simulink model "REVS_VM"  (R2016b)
settings: Solver=ode3  StartTime=REVS.sim_start_time_secs  StopTime=Inf  FixedStep=REVS.sim_step_time_secs  MaxStep=REVS.sim_step_time_secs  EnableMultiTasking=on
StopFcn:
  | postproc_datalog;
  | postproc_audit;
  | postproc_result;
model workspace (MATLAB code in the model file):
  other statements: REVS_setup_variants
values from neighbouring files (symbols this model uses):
  accessory = class_accessory_data    [class_test_data.m]
  battery = class_battery_data    [class_accessory_data.m]    (also in class_REVS_electric.m = class_REVS_battery)
  brake = struct(	'max_torque_Nm',[], 						'proportion_norm',1.0, 						'inertia_kgm2',0.0)    [class_REVS_drive_axle.m]
  engine = class_engine_data    [class_test_data.m]
  final_drive = struct(	'gear_ratio',[], 								'efficiency_norm',[], 								'inertia_kgm2',[] )    [class_REVS_drive_axle.m]
  gear = class_REVS_gearbox    [class_REVS_AT_transmission.m]
  tire = struct(	'radius_m',[], 						'rolling_resistance_coefficient',0, 						'vehicle_weight_norm',1.0,  						'wheel_slip_torque_Nm',[],  						'inertia_kgm2',0.0)    [class_REVS_drive_axle.m]
  torque_converter = class_REVS_torque_converter    [class_REVS_AT_transmission.m]
  transmission = class_transmission_data    [class_test_data.m]
  vehicle = class_vehicle_data    [class_test_data.m]
undefined symbols (not defined in the file or in its folder): alternator, ambient, controls, convert, DelayTimeSecs, drive_cycle, driver, electric, gear_strategy, InitialCondition, InitialValue, LoadSource, LookupStructure, MultiplyPosInputs, Normalize, NumPhases, REVS, SpeedSource, starter, tableshift, UpperSaturationLimit, Value, VerboseLevel, VerboseSignal
libraries: simulink x153
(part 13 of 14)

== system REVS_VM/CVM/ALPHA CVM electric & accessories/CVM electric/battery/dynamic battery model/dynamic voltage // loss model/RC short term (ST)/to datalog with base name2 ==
  Var : Inport
  Constant : Constant  Value=VerboseSignal
  Constant1 : Constant  Value=VerboseLevel
  Relational Operator : RelationalOperator  OutDataTypeStr=boolean  ZeroCross=off
  Subsystem : Subsystem
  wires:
  Constant1/1 -> Relational Operator/2
  Relational Operator/1 -> Subsystem/Enable
  Constant/1 -> Relational Operator/1
  Var/1 -> Subsystem/1(Var)

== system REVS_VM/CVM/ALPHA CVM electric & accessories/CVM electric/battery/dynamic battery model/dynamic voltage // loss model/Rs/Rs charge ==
  bus : Inport
  Bus Selector : BusSelector  OutputSignals=gb.gb_cmd_gear,gb_spd_in_radps,ctrl.gb_line_press_bar
  Lookup : Lookup_n-D  NumberOfTableDimensions=10  BreakpointsForDimension1=LookupStructure.axis_1.breakpoints  BreakpointsForDimension2=LookupStructure.axis_2.breakpoints  BreakpointsForDimension3=LookupStructure.axis_3.breakpoints  BreakpointsForDimension4=LookupStructure.axis_4.breakpoints  BreakpointsForDimension5=LookupStructure.axis_5.breakpoints  BreakpointsForDimension6=LookupStructure.axis_6.breakpoints  BreakpointsForDimension7=LookupStructure.axis_7.breakpoints  BreakpointsForDimension8=LookupStructure.axis_8.breakpoints  BreakpointsForDimension9=LookupStructure.axis_9.breakpoints  BreakpointsForDimension10=LookupStructure.axis_10.breakpoints  IndexSearchMethod=Linear search  BeginIndexSearchUsingPreviousIndexResult=on  Table=LookupStructure.table  InternalRulePriority=Speed  RndMeth=Simplest  SupportTunableTableSize=on  MaximumIndicesForEachDimension=LookupStructure.table_size
  out : Outport
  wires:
  bus/1 -> Bus Selector/1
  Lookup/1 -> out/1

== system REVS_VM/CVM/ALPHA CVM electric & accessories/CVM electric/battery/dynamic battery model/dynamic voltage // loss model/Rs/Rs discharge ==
  bus : Inport
  Bus Selector : BusSelector  OutputSignals=gb.gb_cmd_gear,gb_spd_in_radps,ctrl.gb_line_press_bar
  Lookup : Lookup_n-D  NumberOfTableDimensions=10  BreakpointsForDimension1=LookupStructure.axis_1.breakpoints  BreakpointsForDimension2=LookupStructure.axis_2.breakpoints  BreakpointsForDimension3=LookupStructure.axis_3.breakpoints  BreakpointsForDimension4=LookupStructure.axis_4.breakpoints  BreakpointsForDimension5=LookupStructure.axis_5.breakpoints  BreakpointsForDimension6=LookupStructure.axis_6.breakpoints  BreakpointsForDimension7=LookupStructure.axis_7.breakpoints  BreakpointsForDimension8=LookupStructure.axis_8.breakpoints  BreakpointsForDimension9=LookupStructure.axis_9.breakpoints  BreakpointsForDimension10=LookupStructure.axis_10.breakpoints  IndexSearchMethod=Linear search  BeginIndexSearchUsingPreviousIndexResult=on  Table=LookupStructure.table  InternalRulePriority=Speed  RndMeth=Simplest  SupportTunableTableSize=on  MaximumIndicesForEachDimension=LookupStructure.table_size
  out : Outport
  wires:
  bus/1 -> Bus Selector/1
  Lookup/1 -> out/1

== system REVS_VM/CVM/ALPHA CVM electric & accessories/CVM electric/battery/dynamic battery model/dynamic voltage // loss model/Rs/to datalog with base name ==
  Var : Inport
  Constant : Constant  Value=VerboseSignal
  Constant1 : Constant  Value=VerboseLevel
  Relational Operator : RelationalOperator  OutDataTypeStr=boolean  ZeroCross=off
  Subsystem : Subsystem
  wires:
  Constant1/1 -> Relational Operator/2
  Relational Operator/1 -> Subsystem/Enable
  Constant/1 -> Relational Operator/1
  Var/1 -> Subsystem/1(Var)

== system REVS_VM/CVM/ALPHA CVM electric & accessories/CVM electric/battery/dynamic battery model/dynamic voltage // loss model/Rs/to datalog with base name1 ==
  Var : Inport
  Constant : Constant  Value=VerboseSignal
  Constant1 : Constant  Value=VerboseLevel
  Relational Operator : RelationalOperator  OutDataTypeStr=boolean  ZeroCross=off
  Subsystem : Subsystem
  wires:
  Constant1/1 -> Relational Operator/2
  Relational Operator/1 -> Subsystem/Enable
  Constant/1 -> Relational Operator/1
  Var/1 -> Subsystem/1(Var)

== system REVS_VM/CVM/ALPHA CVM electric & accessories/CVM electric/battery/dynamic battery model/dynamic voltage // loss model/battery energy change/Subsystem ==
  In1 : Inport
  Enable : EnablePort
  To Workspace : ToWorkspace  VariableName=audit__elec__battery__energy_delta_kJ  SampleTime=-1
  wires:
  In1/1 -> To Workspace/1

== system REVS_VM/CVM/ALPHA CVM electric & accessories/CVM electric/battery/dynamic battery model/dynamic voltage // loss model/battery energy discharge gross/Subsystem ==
  In1 : Inport
  Enable : EnablePort
  To Workspace : ToWorkspace  VariableName=audit__elec__battery__discharge_gross_kJ  SampleTime=-1
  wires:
  In1/1 -> To Workspace/1

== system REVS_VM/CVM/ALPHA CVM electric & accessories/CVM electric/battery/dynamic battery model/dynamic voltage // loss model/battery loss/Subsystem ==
  In1 : Inport
  Enable : EnablePort
  To Workspace : ToWorkspace  VariableName=audit__elec__battery__loss_kJ  SampleTime=-1
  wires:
  In1/1 -> To Workspace/1

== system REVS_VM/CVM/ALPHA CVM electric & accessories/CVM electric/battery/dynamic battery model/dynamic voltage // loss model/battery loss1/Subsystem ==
  In1 : Inport
  Enable : EnablePort
  To Workspace : ToWorkspace  VariableName=audit__elec__battery__OCV  SampleTime=-1
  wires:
  In1/1 -> To Workspace/1

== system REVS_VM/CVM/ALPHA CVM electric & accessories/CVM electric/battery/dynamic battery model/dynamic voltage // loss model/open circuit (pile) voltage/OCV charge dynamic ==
  bus : Inport
  Bus Selector : BusSelector  OutputSignals=gb.gb_cmd_gear,gb_spd_in_radps,ctrl.gb_line_press_bar
  Lookup : Lookup_n-D  NumberOfTableDimensions=10  BreakpointsForDimension1=LookupStructure.axis_1.breakpoints  BreakpointsForDimension2=LookupStructure.axis_2.breakpoints  BreakpointsForDimension3=LookupStructure.axis_3.breakpoints  BreakpointsForDimension4=LookupStructure.axis_4.breakpoints  BreakpointsForDimension5=LookupStructure.axis_5.breakpoints  BreakpointsForDimension6=LookupStructure.axis_6.breakpoints  BreakpointsForDimension7=LookupStructure.axis_7.breakpoints  BreakpointsForDimension8=LookupStructure.axis_8.breakpoints  BreakpointsForDimension9=LookupStructure.axis_9.breakpoints  BreakpointsForDimension10=LookupStructure.axis_10.breakpoints  IndexSearchMethod=Linear search  BeginIndexSearchUsingPreviousIndexResult=on  Table=LookupStructure.table  InternalRulePriority=Speed  RndMeth=Simplest  SupportTunableTableSize=on  MaximumIndicesForEachDimension=LookupStructure.table_size
  out : Outport
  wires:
  bus/1 -> Bus Selector/1
  Lookup/1 -> out/1

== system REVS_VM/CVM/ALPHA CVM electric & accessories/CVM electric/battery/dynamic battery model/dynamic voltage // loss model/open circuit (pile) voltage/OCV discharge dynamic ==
  bus : Inport
  Bus Selector : BusSelector  OutputSignals=gb.gb_cmd_gear,gb_spd_in_radps,ctrl.gb_line_press_bar
  Lookup : Lookup_n-D  NumberOfTableDimensions=10  BreakpointsForDimension1=LookupStructure.axis_1.breakpoints  BreakpointsForDimension2=LookupStructure.axis_2.breakpoints  BreakpointsForDimension3=LookupStructure.axis_3.breakpoints  BreakpointsForDimension4=LookupStructure.axis_4.breakpoints  BreakpointsForDimension5=LookupStructure.axis_5.breakpoints  BreakpointsForDimension6=LookupStructure.axis_6.breakpoints  BreakpointsForDimension7=LookupStructure.axis_7.breakpoints  BreakpointsForDimension8=LookupStructure.axis_8.breakpoints  BreakpointsForDimension9=LookupStructure.axis_9.breakpoints  BreakpointsForDimension10=LookupStructure.axis_10.breakpoints  IndexSearchMethod=Linear search  BeginIndexSearchUsingPreviousIndexResult=on  Table=LookupStructure.table  InternalRulePriority=Speed  RndMeth=Simplest  SupportTunableTableSize=on  MaximumIndicesForEachDimension=LookupStructure.table_size
  out : Outport
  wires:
  bus/1 -> Bus Selector/1
  Lookup/1 -> out/1

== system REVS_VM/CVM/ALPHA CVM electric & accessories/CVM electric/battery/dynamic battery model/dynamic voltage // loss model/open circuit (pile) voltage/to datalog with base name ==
  Var : Inport
  Constant : Constant  Value=VerboseSignal
  Constant1 : Constant  Value=VerboseLevel
  Relational Operator : RelationalOperator  OutDataTypeStr=boolean  ZeroCross=off
  Subsystem : Subsystem
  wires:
  Constant1/1 -> Relational Operator/2
  Relational Operator/1 -> Subsystem/Enable
  Constant/1 -> Relational Operator/1
  Var/1 -> Subsystem/1(Var)

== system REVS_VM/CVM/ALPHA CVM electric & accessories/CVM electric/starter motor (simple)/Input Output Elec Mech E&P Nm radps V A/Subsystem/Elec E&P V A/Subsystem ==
  volts_V : Inport
  curr_A : Inport  Port=2
  Enable : EnablePort  ZeroCross=off
  Elec Energy V A : Subsystem  TreatAsAtomicUnit=on
  amps_to_workspace : ToWorkspace  VariableName=audit__elec__starter__input_Amps  SampleTime=-1
  energy_to_workspace : ToWorkspace  VariableName=audit__elec__starter__input_kJ  SampleTime=-1
  neg_energy_to_workspace : ToWorkspace  VariableName=audit__elec__starter__input_neg_kJ  SampleTime=-1
  pos_energy_to_workspace : ToWorkspace  VariableName=audit__elec__starter__input_pos_kJ  SampleTime=-1
  power_to_workspace : ToWorkspace  VariableName=audit__elec__starter__input_kW  SampleTime=-1
  volts_to_workspace : ToWorkspace  VariableName=audit__elec__starter__input_Volts  SampleTime=-1
  pos_kJ : Outport  InitialOutput=0
  neg_kJ : Outport  Port=2  InitialOutput=0
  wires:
  Elec Energy V A/3(neg_kJ) -> neg_kJ/1, neg_energy_to_workspace/1
  Elec Energy V A/4(pwr_kW) -> power_to_workspace/1
  Elec Energy V A/2("pos_kJ ") -> pos_kJ/1, pos_energy_to_workspace/1
  Elec Energy V A/1("total_kJ ") -> energy_to_workspace/1
  volts_V/1 -> volts_to_workspace/1, Elec Energy V A/1(volts_V)
  curr_A/1 -> amps_to_workspace/1, Elec Energy V A/2(curr_A)

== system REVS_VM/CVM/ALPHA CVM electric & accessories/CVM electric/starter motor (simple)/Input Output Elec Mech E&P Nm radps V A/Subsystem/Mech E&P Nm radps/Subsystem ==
  " trq_Nm" : Inport
  spd_radps : Inport  Port=2
  iner_kgm2 : Inport  Port=3
  Enable : EnablePort  ZeroCross=off
  KE_to_workspace : ToWorkspace  VariableName=audit__mech__starter__output_KE_kJ  SampleTime=-1
  Mech Energy Nm radps : Subsystem  TreatAsAtomicUnit=on
  Mult : Product  Inputs=**
  Square : Math  Operator=square
  energy_to_workspace : ToWorkspace  VariableName=audit__mech__starter__output_kJ  SampleTime=-1
  inertia_to_workspace : ToWorkspace  VariableName=audit__mech__starter__output_kgm2  SampleTime=-1
  neg_energy_to_workspace : ToWorkspace  VariableName=audit__mech__starter__output_neg_kJ  SampleTime=-1
  one half : Gain  Gain=0.5/1000
  pos_energy_to_workspace : ToWorkspace  VariableName=audit__mech__starter__output_pos_kJ  SampleTime=-1
  power_to_workspace : ToWorkspace  VariableName=audit__mech__starter__output_kW  SampleTime=-1
  speed_to_workspace : ToWorkspace  VariableName=audit__mech__starter__output_radps  SampleTime=-1
  torque_to_workspace : ToWorkspace  VariableName=audit__mech__starter__output_Nm  SampleTime=-1
  pos_kJ : Outport  InitialOutput=0
  neg_kJ : Outport  Port=2  InitialOutput=0
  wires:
  Mult/1 -> one half/1
  Square/1 -> Mult/1
  one half/1 -> KE_to_workspace/1
  Mech Energy Nm radps/4(pwr_kW) -> power_to_workspace/1
  Mech Energy Nm radps/1("total_kJ ") -> energy_to_workspace/1
  iner_kgm2/1 -> inertia_to_workspace/1, Mult/2
  spd_radps/1 -> Mech Energy Nm radps/2(spd_radps), speed_to_workspace/1, Square/1
  " trq_Nm"/1 -> Mech Energy Nm radps/1(trq_Nm), torque_to_workspace/1
  Mech Energy Nm radps/2("pos_kJ ") -> pos_kJ/1, pos_energy_to_workspace/1
  Mech Energy Nm radps/3(neg_kJ) -> neg_energy_to_workspace/1, neg_kJ/1

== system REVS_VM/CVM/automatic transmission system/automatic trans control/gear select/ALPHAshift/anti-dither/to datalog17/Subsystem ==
  In1 : Inport
  Enable : EnablePort
  To Workspace : ToWorkspace  VariableName=datalog__ALPHAshift__filtered_desired_gear_num  SampleTime=-1
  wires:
  In1/1 -> To Workspace/1

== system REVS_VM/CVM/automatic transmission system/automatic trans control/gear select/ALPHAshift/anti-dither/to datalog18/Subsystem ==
  In1 : Inport
  Enable : EnablePort
  To Workspace : ToWorkspace  VariableName=datalog__ALPHAshift__raw_desired_gear_num  SampleTime=-1
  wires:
  In1/1 -> To Workspace/1

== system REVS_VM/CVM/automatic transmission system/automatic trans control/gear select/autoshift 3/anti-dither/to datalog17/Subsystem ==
  In1 : Inport
  Enable : EnablePort
  To Workspace : ToWorkspace  VariableName=datalog__autoshift3__filtered_desired_gear_num  SampleTime=-1
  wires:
  In1/1 -> To Workspace/1

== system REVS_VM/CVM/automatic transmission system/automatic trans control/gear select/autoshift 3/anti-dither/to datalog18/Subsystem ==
  In1 : Inport
  Enable : EnablePort
  To Workspace : ToWorkspace  VariableName=datalog__autoshift3__raw_desired_gear_num  SampleTime=-1
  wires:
  In1/1 -> To Workspace/1

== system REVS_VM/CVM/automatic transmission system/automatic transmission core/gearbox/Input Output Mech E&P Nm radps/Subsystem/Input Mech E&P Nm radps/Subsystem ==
  " trq_Nm" : Inport
  spd_radps : Inport  Port=2
  iner_kgm2 : Inport  Port=3
  Enable : EnablePort  ZeroCross=off
  KE_to_workspace : ToWorkspace  VariableName=audit__mech__gearbox__input_KE_kJ  SampleTime=-1
  Mech Energy Nm radps : Subsystem  TreatAsAtomicUnit=on
  Mult : Product  Inputs=**
  Square : Math  Operator=square
  energy_to_workspace : ToWorkspace  VariableName=audit__mech__gearbox__input_kJ  SampleTime=-1
  inertia_to_workspace : ToWorkspace  VariableName=audit__mech__gearbox__input_kgm2  SampleTime=-1
  neg_energy_to_workspace : ToWorkspace  VariableName=audit__mech__gearbox__input_neg_kJ  SampleTime=-1
  one half : Gain  Gain=0.5/1000
  pos_energy_to_workspace : ToWorkspace  VariableName=audit__mech__gearbox__input_pos_kJ  SampleTime=-1
  power_to_workspace : ToWorkspace  VariableName=audit__mech__gearbox__input_kW  SampleTime=-1
  speed_to_workspace : ToWorkspace  VariableName=audit__mech__gearbox__input_radps  SampleTime=-1
  torque_to_workspace : ToWorkspace  VariableName=audit__mech__gearbox__input_Nm  SampleTime=-1
  pos_kJ : Outport  InitialOutput=0
  neg_kJ : Outport  Port=2  InitialOutput=0
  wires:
  Mult/1 -> one half/1
  Square/1 -> Mult/1
  one half/1 -> KE_to_workspace/1
  Mech Energy Nm radps/4(pwr_kW) -> power_to_workspace/1
  Mech Energy Nm radps/1("total_kJ ") -> energy_to_workspace/1
  iner_kgm2/1 -> inertia_to_workspace/1, Mult/2
  spd_radps/1 -> Mech Energy Nm radps/2(spd_radps), speed_to_workspace/1, Square/1
  " trq_Nm"/1 -> Mech Energy Nm radps/1(trq_Nm), torque_to_workspace/1
  Mech Energy Nm radps/2("pos_kJ ") -> pos_kJ/1, pos_energy_to_workspace/1
  Mech Energy Nm radps/3(neg_kJ) -> neg_energy_to_workspace/1, neg_kJ/1

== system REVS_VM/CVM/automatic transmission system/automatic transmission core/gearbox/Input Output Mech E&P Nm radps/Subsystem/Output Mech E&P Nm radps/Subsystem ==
  " trq_Nm" : Inport
  spd_radps : Inport  Port=2
  iner_kgm2 : Inport  Port=3
  Enable : EnablePort  ZeroCross=off
  KE_to_workspace : ToWorkspace  VariableName=audit__mech__gearbox__output_KE_kJ  SampleTime=-1
  Mech Energy Nm radps : Subsystem  TreatAsAtomicUnit=on
  Mult : Product  Inputs=**
  Square : Math  Operator=square
  energy_to_workspace : ToWorkspace  VariableName=audit__mech__gearbox__output_kJ  SampleTime=-1
  inertia_to_workspace : ToWorkspace  VariableName=audit__mech__gearbox__output_kgm2  SampleTime=-1
  neg_energy_to_workspace : ToWorkspace  VariableName=audit__mech__gearbox__output_neg_kJ  SampleTime=-1
  one half : Gain  Gain=0.5/1000
  pos_energy_to_workspace : ToWorkspace  VariableName=audit__mech__gearbox__output_pos_kJ  SampleTime=-1
  power_to_workspace : ToWorkspace  VariableName=audit__mech__gearbox__output_kW  SampleTime=-1
  speed_to_workspace : ToWorkspace  VariableName=audit__mech__gearbox__output_radps  SampleTime=-1
  torque_to_workspace : ToWorkspace  VariableName=audit__mech__gearbox__output_Nm  SampleTime=-1
  pos_kJ : Outport  InitialOutput=0
  neg_kJ : Outport  Port=2  InitialOutput=0
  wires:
  Mult/1 -> one half/1
  Square/1 -> Mult/1
  one half/1 -> KE_to_workspace/1
  Mech Energy Nm radps/4(pwr_kW) -> power_to_workspace/1
  Mech Energy Nm radps/1("total_kJ ") -> energy_to_workspace/1
  iner_kgm2/1 -> inertia_to_workspace/1, Mult/2
  spd_radps/1 -> Mech Energy Nm radps/2(spd_radps), speed_to_workspace/1, Square/1
  " trq_Nm"/1 -> Mech Energy Nm radps/1(trq_Nm), torque_to_workspace/1
  Mech Energy Nm radps/2("pos_kJ ") -> pos_kJ/1, pos_energy_to_workspace/1
  Mech Energy Nm radps/3(neg_kJ) -> neg_energy_to_workspace/1, neg_kJ/1

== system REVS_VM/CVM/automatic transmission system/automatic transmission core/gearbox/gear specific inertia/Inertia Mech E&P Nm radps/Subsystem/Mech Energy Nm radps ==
  trq_Nm : Inport
  spd_radps : Inport  Port=2
  Gain : Gain  Gain=-1
  Integrator : Integrator  ZeroCross=off
  Integrator1 : Integrator  ZeroCross=off
  Integrator2 : Integrator  ZeroCross=off
  Mux : Mux  Inputs=2
  Neg : Fcn  Expr=u(1)*(u(1) <= 0)
  Pos : Fcn  Expr=u(1)*(u(1) >= 0)
  calc_Power_kW : Fcn  Expr=u(1)*u(2)/1000
  "total_kJ " : Outport
  "pos_kJ " : Outport  Port=2
  neg_kJ : Outport  Port=3
  pwr_kW : Outport  Port=4
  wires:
  calc_Power_kW/1 -> Pos/1, Neg/1, pwr_kW/1, Integrator/1
  Gain/1 -> neg_kJ/1
  Integrator1/1 -> "pos_kJ "/1
  Integrator2/1 -> Gain/1
  Neg/1 -> Integrator2/1
  Pos/1 -> Integrator1/1
  spd_radps/1 -> Mux/2
  trq_Nm/1 -> Mux/1
  Mux/1 -> calc_Power_kW/1
  Integrator/1 -> "total_kJ "/1

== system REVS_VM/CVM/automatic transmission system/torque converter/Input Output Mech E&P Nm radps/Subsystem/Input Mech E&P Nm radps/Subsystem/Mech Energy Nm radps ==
  trq_Nm : Inport
  spd_radps : Inport  Port=2
  Gain : Gain  Gain=-1
  Integrator : Integrator  ZeroCross=off
  Integrator1 : Integrator  ZeroCross=off
  Integrator2 : Integrator  ZeroCross=off
  Mux : Mux  Inputs=2
  Neg : Fcn  Expr=u(1)*(u(1) <= 0)
  Pos : Fcn  Expr=u(1)*(u(1) >= 0)
  calc_Power_kW : Fcn  Expr=u(1)*u(2)/1000
  "total_kJ " : Outport
  "pos_kJ " : Outport  Port=2
  neg_kJ : Outport  Port=3
  pwr_kW : Outport  Port=4
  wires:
  calc_Power_kW/1 -> Pos/1, Neg/1, pwr_kW/1, Integrator/1
  Gain/1 -> neg_kJ/1
  Integrator1/1 -> "pos_kJ "/1
  Integrator2/1 -> Gain/1
  Neg/1 -> Integrator2/1
  Pos/1 -> Integrator1/1
  spd_radps/1 -> Mux/2
  trq_Nm/1 -> Mux/1
  Mux/1 -> calc_Power_kW/1
  Integrator/1 -> "total_kJ "/1

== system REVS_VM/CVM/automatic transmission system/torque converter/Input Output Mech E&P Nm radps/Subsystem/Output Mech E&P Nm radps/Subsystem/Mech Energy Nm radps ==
  trq_Nm : Inport
  spd_radps : Inport  Port=2
  Gain : Gain  Gain=-1
  Integrator : Integrator  ZeroCross=off
  Integrator1 : Integrator  ZeroCross=off
  Integrator2 : Integrator  ZeroCross=off
  Mux : Mux  Inputs=2
  Neg : Fcn  Expr=u(1)*(u(1) <= 0)
  Pos : Fcn  Expr=u(1)*(u(1) >= 0)
  calc_Power_kW : Fcn  Expr=u(1)*u(2)/1000
  "total_kJ " : Outport
  "pos_kJ " : Outport  Port=2
  neg_kJ : Outport  Port=3
  pwr_kW : Outport  Port=4
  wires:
  calc_Power_kW/1 -> Pos/1, Neg/1, pwr_kW/1, Integrator/1
  Gain/1 -> neg_kJ/1
  Integrator1/1 -> "pos_kJ "/1
  Integrator2/1 -> Gain/1
  Neg/1 -> Integrator2/1
  Pos/1 -> Integrator1/1
  spd_radps/1 -> Mux/2
  trq_Nm/1 -> Mux/1
  Mux/1 -> calc_Power_kW/1
  Integrator/1 -> "total_kJ "/1

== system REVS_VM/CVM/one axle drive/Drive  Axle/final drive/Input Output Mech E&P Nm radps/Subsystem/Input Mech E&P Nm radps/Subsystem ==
  " trq_Nm" : Inport
  spd_radps : Inport  Port=2
  iner_kgm2 : Inport  Port=3
  Enable : EnablePort  ZeroCross=off
  KE_to_workspace : ToWorkspace  VariableName=audit__mech__drive_axle1__final_drive__input_KE_kJ  SampleTime=-1
  Mech Energy Nm radps : Subsystem  TreatAsAtomicUnit=on
  Mult : Product  Inputs=**
  Square : Math  Operator=square
  energy_to_workspace : ToWorkspace  VariableName=audit__mech__drive_axle1__final_drive__input_kJ  SampleTime=-1
  inertia_to_workspace : ToWorkspace  VariableName=audit__mech__drive_axle1__final_drive__input_kgm2  SampleTime=-1
  neg_energy_to_workspace : ToWorkspace  VariableName=audit__mech__drive_axle1__final_drive__input_neg_kJ  SampleTime=-1
  one half : Gain  Gain=0.5/1000
  pos_energy_to_workspace : ToWorkspace  VariableName=audit__mech__drive_axle1__final_drive__input_pos_kJ  SampleTime=-1
  power_to_workspace : ToWorkspace  VariableName=audit__mech__drive_axle1__final_drive__input_kW  SampleTime=-1
  speed_to_workspace : ToWorkspace  VariableName=audit__mech__drive_axle1__final_drive__input_radps  SampleTime=-1
  torque_to_workspace : ToWorkspace  VariableName=audit__mech__drive_axle1__final_drive__input_Nm  SampleTime=-1
  pos_kJ : Outport  InitialOutput=0
  neg_kJ : Outport  Port=2  InitialOutput=0
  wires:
  Mult/1 -> one half/1
  Square/1 -> Mult/1
  one half/1 -> KE_to_workspace/1
  Mech Energy Nm radps/4(pwr_kW) -> power_to_workspace/1
  Mech Energy Nm radps/1("total_kJ ") -> energy_to_workspace/1
  iner_kgm2/1 -> inertia_to_workspace/1, Mult/2
  spd_radps/1 -> Mech Energy Nm radps/2(spd_radps), speed_to_workspace/1, Square/1
  " trq_Nm"/1 -> Mech Energy Nm radps/1(trq_Nm), torque_to_workspace/1
  Mech Energy Nm radps/2("pos_kJ ") -> pos_kJ/1, pos_energy_to_workspace/1
  Mech Energy Nm radps/3(neg_kJ) -> neg_energy_to_workspace/1, neg_kJ/1

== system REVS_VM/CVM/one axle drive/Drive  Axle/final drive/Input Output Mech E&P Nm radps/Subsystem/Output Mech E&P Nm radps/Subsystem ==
  " trq_Nm" : Inport
  spd_radps : Inport  Port=2
  iner_kgm2 : Inport  Port=3
  Enable : EnablePort  ZeroCross=off
  KE_to_workspace : ToWorkspace  VariableName=audit__mech__drive_axle1__final_drive__output_KE_kJ  SampleTime=-1
  Mech Energy Nm radps : Subsystem  TreatAsAtomicUnit=on
  Mult : Product  Inputs=**
  Square : Math  Operator=square
  energy_to_workspace : ToWorkspace  VariableName=audit__mech__drive_axle1__final_drive__output_kJ  SampleTime=-1
  inertia_to_workspace : ToWorkspace  VariableName=audit__mech__drive_axle1__final_drive__output_kgm2  SampleTime=-1
  neg_energy_to_workspace : ToWorkspace  VariableName=audit__mech__drive_axle1__final_drive__output_neg_kJ  SampleTime=-1
  one half : Gain  Gain=0.5/1000
  pos_energy_to_workspace : ToWorkspace  VariableName=audit__mech__drive_axle1__final_drive__output_pos_kJ  SampleTime=-1
  power_to_workspace : ToWorkspace  VariableName=audit__mech__drive_axle1__final_drive__output_kW  SampleTime=-1
  speed_to_workspace : ToWorkspace  VariableName=audit__mech__drive_axle1__final_drive__output_radps  SampleTime=-1
  torque_to_workspace : ToWorkspace  VariableName=audit__mech__drive_axle1__final_drive__output_Nm  SampleTime=-1
  pos_kJ : Outport  InitialOutput=0
  neg_kJ : Outport  Port=2  InitialOutput=0
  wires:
  Mult/1 -> one half/1
  Square/1 -> Mult/1
  one half/1 -> KE_to_workspace/1
  Mech Energy Nm radps/4(pwr_kW) -> power_to_workspace/1
  Mech Energy Nm radps/1("total_kJ ") -> energy_to_workspace/1
  iner_kgm2/1 -> inertia_to_workspace/1, Mult/2
  spd_radps/1 -> Mech Energy Nm radps/2(spd_radps), speed_to_workspace/1, Square/1
  " trq_Nm"/1 -> Mech Energy Nm radps/1(trq_Nm), torque_to_workspace/1
  Mech Energy Nm radps/2("pos_kJ ") -> pos_kJ/1, pos_energy_to_workspace/1
  Mech Energy Nm radps/3(neg_kJ) -> neg_energy_to_workspace/1, neg_kJ/1

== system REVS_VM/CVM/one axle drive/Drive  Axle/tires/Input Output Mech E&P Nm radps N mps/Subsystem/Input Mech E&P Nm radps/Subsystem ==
  " trq_Nm" : Inport
  spd_radps : Inport  Port=2
  iner_kgm2 : Inport  Port=3
  Enable : EnablePort  ZeroCross=off
  KE_to_workspace : ToWorkspace  VariableName=audit__mech__drive_axle1__tire__input_KE_kJ  SampleTime=-1
  Mech Energy Nm radps : Subsystem  TreatAsAtomicUnit=on
  Mult : Product  Inputs=**
  Square : Math  Operator=square
  energy_to_workspace : ToWorkspace  VariableName=audit__mech__drive_axle1__tire__input_kJ  SampleTime=-1
  inertia_to_workspace : ToWorkspace  VariableName=audit__mech__drive_axle1__tire__input_kgm2  SampleTime=-1
  neg_energy_to_workspace : ToWorkspace  VariableName=audit__mech__drive_axle1__tire__input_neg_kJ  SampleTime=-1
  one half : Gain  Gain=0.5/1000
  pos_energy_to_workspace : ToWorkspace  VariableName=audit__mech__drive_axle1__tire__input_pos_kJ  SampleTime=-1
  power_to_workspace : ToWorkspace  VariableName=audit__mech__drive_axle1__tire__input_kW  SampleTime=-1
  speed_to_workspace : ToWorkspace  VariableName=audit__mech__drive_axle1__tire__input_radps  SampleTime=-1
  torque_to_workspace : ToWorkspace  VariableName=audit__mech__drive_axle1__tire__input_Nm  SampleTime=-1
  pos_kJ : Outport  InitialOutput=0
  neg_kJ : Outport  Port=2  InitialOutput=0
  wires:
  Mech Energy Nm radps/3(neg_kJ) -> neg_kJ/1, neg_energy_to_workspace/1
  Mech Energy Nm radps/2("pos_kJ ") -> pos_energy_to_workspace/1, pos_kJ/1
  " trq_Nm"/1 -> torque_to_workspace/1, Mech Energy Nm radps/1(trq_Nm)
  spd_radps/1 -> Square/1, speed_to_workspace/1, Mech Energy Nm radps/2(spd_radps)
  iner_kgm2/1 -> Mult/2, inertia_to_workspace/1
  Mech Energy Nm radps/1("total_kJ ") -> energy_to_workspace/1
  Mech Energy Nm radps/4(pwr_kW) -> power_to_workspace/1
  one half/1 -> KE_to_workspace/1
  Square/1 -> Mult/1
  Mult/1 -> one half/1

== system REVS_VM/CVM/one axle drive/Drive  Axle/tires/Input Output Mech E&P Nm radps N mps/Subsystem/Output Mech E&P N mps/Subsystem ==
  force_N : Inport
  spd_mps : Inport  Port=2
  mass_kg : Inport  Port=3
  Enable : EnablePort  ZeroCross=off
  Integrator1 : Integrator  LimitOutput=on  UpperSaturationLimit=Inf  LowerSaturationLimit=0  ZeroCross=off
  KE_to_workspace : ToWorkspace  VariableName=audit__mech__drive_axle1__tire__output_KE_kJ  SampleTime=-1
  Mech Energy N mps : Subsystem  TreatAsAtomicUnit=on
  Mult : Product  Inputs=**
  Square : Math  Operator=square
  distance_to_workspace : ToWorkspace  VariableName=audit__mech__drive_axle1__tire__output_m  SampleTime=-1
  energy_to_workspace : ToWorkspace  VariableName=audit__mech__drive_axle1__tire__output_kJ  SampleTime=-1
  force_to_workspace : ToWorkspace  VariableName=audit__mech__drive_axle1__tire__output_N  SampleTime=-1
  mass_to_workspace : ToWorkspace  VariableName=audit__mech__drive_axle1__tire__output_kg  SampleTime=-1
  neg_energy_to_workspace : ToWorkspace  VariableName=audit__mech__drive_axle1__tire__output_neg_kJ  SampleTime=-1
  one half : Gain  Gain=0.5/1000
  pos_energy_to_workspace : ToWorkspace  VariableName=audit__mech__drive_axle1__tire__output_pos_kJ  SampleTime=-1
  power_to_workspace : ToWorkspace  VariableName=audit__mech__drive_axle1__tire__output_kW  SampleTime=-1
  speed_to_workspace : ToWorkspace  VariableName=audit__mech__drive_axle1__tire__output_mps  SampleTime=-1
  pos_kJ : Outport
  neg_kJ : Outport  Port=2
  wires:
  Mech Energy N mps/3(neg_kJ) -> neg_energy_to_workspace/1, neg_kJ/1
  Mech Energy N mps/2("pos_kJ ") -> pos_energy_to_workspace/1, pos_kJ/1
  Mech Energy N mps/1("total_kJ ") -> energy_to_workspace/1
  Mech Energy N mps/4(pwr_kW) -> power_to_workspace/1
  one half/1 -> KE_to_workspace/1
  Square/1 -> Mult/1
  Mult/1 -> one half/1
  mass_kg/1 -> Mult/2, mass_to_workspace/1
  spd_mps/1 -> Mech Energy N mps/2(spd_mps), Integrator1/1, Square/1, speed_to_workspace/1
  force_N/1 -> Mech Energy N mps/1(force_N), force_to_workspace/1
  Integrator1/1 -> distance_to_workspace/1

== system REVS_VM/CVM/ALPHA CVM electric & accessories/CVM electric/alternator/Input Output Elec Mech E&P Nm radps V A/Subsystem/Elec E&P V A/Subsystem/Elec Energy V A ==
  volts_V : Inport
  curr_A : Inport  Port=2
  Gain : Gain  Gain=-1
  Integrator : Integrator  ZeroCross=off
  Integrator1 : Integrator  ZeroCross=off
  Integrator2 : Integrator  ZeroCross=off
  Mux : Mux  Inputs=2
  Neg : Fcn  Expr=u(1)*(u(1) <= 0)
  Pos : Fcn  Expr=u(1)*(u(1) >= 0)
  calc_Power_kW : Fcn  Expr=u(1)*u(2)/1000
  "total_kJ " : Outport
  "pos_kJ " : Outport  Port=2
  neg_kJ : Outport  Port=3
  pwr_kW : Outport  Port=4
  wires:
  curr_A/1 -> Mux/2
  volts_V/1 -> Mux/1
  Mux/1 -> calc_Power_kW/1
  Integrator/1 -> "total_kJ "/1
  Pos/1 -> Integrator1/1
  Neg/1 -> Integrator2/1
  Integrator2/1 -> Gain/1
  Integrator1/1 -> "pos_kJ "/1
  Gain/1 -> neg_kJ/1
  calc_Power_kW/1 -> Integrator/1, pwr_kW/1, Neg/1, Pos/1

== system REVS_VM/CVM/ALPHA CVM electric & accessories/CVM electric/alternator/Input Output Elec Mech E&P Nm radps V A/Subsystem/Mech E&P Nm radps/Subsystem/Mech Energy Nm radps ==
  trq_Nm : Inport
  spd_radps : Inport  Port=2
  Gain : Gain  Gain=-1
  Integrator : Integrator  ZeroCross=off
  Integrator1 : Integrator  ZeroCross=off
  Integrator2 : Integrator  ZeroCross=off
  Mux : Mux  Inputs=2
  Neg : Fcn  Expr=u(1)*(u(1) <= 0)
  Pos : Fcn  Expr=u(1)*(u(1) >= 0)
  calc_Power_kW : Fcn  Expr=u(1)*u(2)/1000
  "total_kJ " : Outport
  "pos_kJ " : Outport  Port=2
  neg_kJ : Outport  Port=3
  pwr_kW : Outport  Port=4
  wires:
  calc_Power_kW/1 -> Pos/1, Neg/1, pwr_kW/1, Integrator/1
  Gain/1 -> neg_kJ/1
  Integrator1/1 -> "pos_kJ "/1
  Integrator2/1 -> Gain/1
  Neg/1 -> Integrator2/1
  Pos/1 -> Integrator1/1
  spd_radps/1 -> Mux/2
  trq_Nm/1 -> Mux/1
  Mux/1 -> calc_Power_kW/1
  Integrator/1 -> "total_kJ "/1

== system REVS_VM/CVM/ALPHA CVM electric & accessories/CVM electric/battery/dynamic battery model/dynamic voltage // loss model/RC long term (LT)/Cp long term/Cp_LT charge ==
  bus : Inport
  Bus Selector : BusSelector  OutputSignals=gb.gb_cmd_gear,gb_spd_in_radps,ctrl.gb_line_press_bar
  Lookup : Lookup_n-D  NumberOfTableDimensions=10  BreakpointsForDimension1=LookupStructure.axis_1.breakpoints  BreakpointsForDimension2=LookupStructure.axis_2.breakpoints  BreakpointsForDimension3=LookupStructure.axis_3.breakpoints  BreakpointsForDimension4=LookupStructure.axis_4.breakpoints  BreakpointsForDimension5=LookupStructure.axis_5.breakpoints  BreakpointsForDimension6=LookupStructure.axis_6.breakpoints  BreakpointsForDimension7=LookupStructure.axis_7.breakpoints  BreakpointsForDimension8=LookupStructure.axis_8.breakpoints  BreakpointsForDimension9=LookupStructure.axis_9.breakpoints  BreakpointsForDimension10=LookupStructure.axis_10.breakpoints  IndexSearchMethod=Linear search  BeginIndexSearchUsingPreviousIndexResult=on  Table=LookupStructure.table  InternalRulePriority=Speed  RndMeth=Simplest  SupportTunableTableSize=on  MaximumIndicesForEachDimension=LookupStructure.table_size
  out : Outport
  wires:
  bus/1 -> Bus Selector/1
  Lookup/1 -> out/1

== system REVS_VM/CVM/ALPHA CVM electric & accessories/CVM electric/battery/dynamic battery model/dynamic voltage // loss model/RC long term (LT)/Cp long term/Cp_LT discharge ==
  bus : Inport
  Bus Selector : BusSelector  OutputSignals=gb.gb_cmd_gear,gb_spd_in_radps,ctrl.gb_line_press_bar
  Lookup : Lookup_n-D  NumberOfTableDimensions=10  BreakpointsForDimension1=LookupStructure.axis_1.breakpoints  BreakpointsForDimension2=LookupStructure.axis_2.breakpoints  BreakpointsForDimension3=LookupStructure.axis_3.breakpoints  BreakpointsForDimension4=LookupStructure.axis_4.breakpoints  BreakpointsForDimension5=LookupStructure.axis_5.breakpoints  BreakpointsForDimension6=LookupStructure.axis_6.breakpoints  BreakpointsForDimension7=LookupStructure.axis_7.breakpoints  BreakpointsForDimension8=LookupStructure.axis_8.breakpoints  BreakpointsForDimension9=LookupStructure.axis_9.breakpoints  BreakpointsForDimension10=LookupStructure.axis_10.breakpoints  IndexSearchMethod=Linear search  BeginIndexSearchUsingPreviousIndexResult=on  Table=LookupStructure.table  InternalRulePriority=Speed  RndMeth=Simplest  SupportTunableTableSize=on  MaximumIndicesForEachDimension=LookupStructure.table_size
  out : Outport
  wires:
  bus/1 -> Bus Selector/1
  Lookup/1 -> out/1

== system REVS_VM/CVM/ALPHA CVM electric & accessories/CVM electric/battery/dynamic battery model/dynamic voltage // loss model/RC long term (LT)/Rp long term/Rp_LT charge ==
  bus : Inport
  Bus Selector : BusSelector  OutputSignals=gb.gb_cmd_gear,gb_spd_in_radps,ctrl.gb_line_press_bar
  Lookup : Lookup_n-D  NumberOfTableDimensions=10  BreakpointsForDimension1=LookupStructure.axis_1.breakpoints  BreakpointsForDimension2=LookupStructure.axis_2.breakpoints  BreakpointsForDimension3=LookupStructure.axis_3.breakpoints  BreakpointsForDimension4=LookupStructure.axis_4.breakpoints  BreakpointsForDimension5=LookupStructure.axis_5.breakpoints  BreakpointsForDimension6=LookupStructure.axis_6.breakpoints  BreakpointsForDimension7=LookupStructure.axis_7.breakpoints  BreakpointsForDimension8=LookupStructure.axis_8.breakpoints  BreakpointsForDimension9=LookupStructure.axis_9.breakpoints  BreakpointsForDimension10=LookupStructure.axis_10.breakpoints  IndexSearchMethod=Linear search  BeginIndexSearchUsingPreviousIndexResult=on  Table=LookupStructure.table  InternalRulePriority=Speed  RndMeth=Simplest  SupportTunableTableSize=on  MaximumIndicesForEachDimension=LookupStructure.table_size
  out : Outport
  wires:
  bus/1 -> Bus Selector/1
  Lookup/1 -> out/1

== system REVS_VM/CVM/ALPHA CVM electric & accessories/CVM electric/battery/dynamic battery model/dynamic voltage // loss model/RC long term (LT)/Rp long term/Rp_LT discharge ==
  bus : Inport
  Bus Selector : BusSelector  OutputSignals=gb.gb_cmd_gear,gb_spd_in_radps,ctrl.gb_line_press_bar
  Lookup : Lookup_n-D  NumberOfTableDimensions=10  BreakpointsForDimension1=LookupStructure.axis_1.breakpoints  BreakpointsForDimension2=LookupStructure.axis_2.breakpoints  BreakpointsForDimension3=LookupStructure.axis_3.breakpoints  BreakpointsForDimension4=LookupStructure.axis_4.breakpoints  BreakpointsForDimension5=LookupStructure.axis_5.breakpoints  BreakpointsForDimension6=LookupStructure.axis_6.breakpoints  BreakpointsForDimension7=LookupStructure.axis_7.breakpoints  BreakpointsForDimension8=LookupStructure.axis_8.breakpoints  BreakpointsForDimension9=LookupStructure.axis_9.breakpoints  BreakpointsForDimension10=LookupStructure.axis_10.breakpoints  IndexSearchMethod=Linear search  BeginIndexSearchUsingPreviousIndexResult=on  Table=LookupStructure.table  InternalRulePriority=Speed  RndMeth=Simplest  SupportTunableTableSize=on  MaximumIndicesForEachDimension=LookupStructure.table_size
  out : Outport
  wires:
  bus/1 -> Bus Selector/1
  Lookup/1 -> out/1

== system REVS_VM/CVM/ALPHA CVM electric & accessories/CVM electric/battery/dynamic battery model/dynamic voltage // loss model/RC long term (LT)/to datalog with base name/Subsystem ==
  Var : Inport
  Enable : EnablePort
  To Workspace : ToWorkspace  VariableName=datalog__battery__RC_LT_V  SampleTime=-1
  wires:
  Var/1 -> To Workspace/1

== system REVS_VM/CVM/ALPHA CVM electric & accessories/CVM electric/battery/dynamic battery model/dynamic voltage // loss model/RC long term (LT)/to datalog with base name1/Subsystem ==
  Var : Inport
  Enable : EnablePort
  To Workspace : ToWorkspace  VariableName=datalog__battery__RC_LT_Ohm  SampleTime=-1
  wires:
  Var/1 -> To Workspace/1

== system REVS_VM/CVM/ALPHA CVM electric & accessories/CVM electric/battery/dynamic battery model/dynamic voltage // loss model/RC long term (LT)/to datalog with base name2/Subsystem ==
  Var : Inport
  Enable : EnablePort
  To Workspace : ToWorkspace  VariableName=datalog__battery__RC_LT_Farad  SampleTime=-1
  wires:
  Var/1 -> To Workspace/1

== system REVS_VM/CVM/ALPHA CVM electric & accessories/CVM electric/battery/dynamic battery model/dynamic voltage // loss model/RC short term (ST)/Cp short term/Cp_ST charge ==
  bus : Inport
  Bus Selector : BusSelector  OutputSignals=gb.gb_cmd_gear,gb_spd_in_radps,ctrl.gb_line_press_bar
  Lookup : Lookup_n-D  NumberOfTableDimensions=10  BreakpointsForDimension1=LookupStructure.axis_1.breakpoints  BreakpointsForDimension2=LookupStructure.axis_2.breakpoints  BreakpointsForDimension3=LookupStructure.axis_3.breakpoints  BreakpointsForDimension4=LookupStructure.axis_4.breakpoints  BreakpointsForDimension5=LookupStructure.axis_5.breakpoints  BreakpointsForDimension6=LookupStructure.axis_6.breakpoints  BreakpointsForDimension7=LookupStructure.axis_7.breakpoints  BreakpointsForDimension8=LookupStructure.axis_8.breakpoints  BreakpointsForDimension9=LookupStructure.axis_9.breakpoints  BreakpointsForDimension10=LookupStructure.axis_10.breakpoints  IndexSearchMethod=Linear search  BeginIndexSearchUsingPreviousIndexResult=on  Table=LookupStructure.table  InternalRulePriority=Speed  RndMeth=Simplest  SupportTunableTableSize=on  MaximumIndicesForEachDimension=LookupStructure.table_size
  out : Outport
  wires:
  bus/1 -> Bus Selector/1
  Lookup/1 -> out/1

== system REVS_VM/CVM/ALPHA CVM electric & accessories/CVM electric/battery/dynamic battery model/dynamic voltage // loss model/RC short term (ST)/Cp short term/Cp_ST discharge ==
  bus : Inport
  Bus Selector : BusSelector  OutputSignals=gb.gb_cmd_gear,gb_spd_in_radps,ctrl.gb_line_press_bar
  Lookup : Lookup_n-D  NumberOfTableDimensions=10  BreakpointsForDimension1=LookupStructure.axis_1.breakpoints  BreakpointsForDimension2=LookupStructure.axis_2.breakpoints  BreakpointsForDimension3=LookupStructure.axis_3.breakpoints  BreakpointsForDimension4=LookupStructure.axis_4.breakpoints  BreakpointsForDimension5=LookupStructure.axis_5.breakpoints  BreakpointsForDimension6=LookupStructure.axis_6.breakpoints  BreakpointsForDimension7=LookupStructure.axis_7.breakpoints  BreakpointsForDimension8=LookupStructure.axis_8.breakpoints  BreakpointsForDimension9=LookupStructure.axis_9.breakpoints  BreakpointsForDimension10=LookupStructure.axis_10.breakpoints  IndexSearchMethod=Linear search  BeginIndexSearchUsingPreviousIndexResult=on  Table=LookupStructure.table  InternalRulePriority=Speed  RndMeth=Simplest  SupportTunableTableSize=on  MaximumIndicesForEachDimension=LookupStructure.table_size
  out : Outport
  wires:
  bus/1 -> Bus Selector/1
  Lookup/1 -> out/1

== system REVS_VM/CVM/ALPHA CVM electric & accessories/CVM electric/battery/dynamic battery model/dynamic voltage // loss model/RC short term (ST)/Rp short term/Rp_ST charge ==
  bus : Inport
  Bus Selector : BusSelector  OutputSignals=gb.gb_cmd_gear,gb_spd_in_radps,ctrl.gb_line_press_bar
  Lookup : Lookup_n-D  NumberOfTableDimensions=10  BreakpointsForDimension1=LookupStructure.axis_1.breakpoints  BreakpointsForDimension2=LookupStructure.axis_2.breakpoints  BreakpointsForDimension3=LookupStructure.axis_3.breakpoints  BreakpointsForDimension4=LookupStructure.axis_4.breakpoints  BreakpointsForDimension5=LookupStructure.axis_5.breakpoints  BreakpointsForDimension6=LookupStructure.axis_6.breakpoints  BreakpointsForDimension7=LookupStructure.axis_7.breakpoints  BreakpointsForDimension8=LookupStructure.axis_8.breakpoints  BreakpointsForDimension9=LookupStructure.axis_9.breakpoints  BreakpointsForDimension10=LookupStructure.axis_10.breakpoints  IndexSearchMethod=Linear search  BeginIndexSearchUsingPreviousIndexResult=on  Table=LookupStructure.table  InternalRulePriority=Speed  RndMeth=Simplest  SupportTunableTableSize=on  MaximumIndicesForEachDimension=LookupStructure.table_size
  out : Outport
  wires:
  bus/1 -> Bus Selector/1
  Lookup/1 -> out/1

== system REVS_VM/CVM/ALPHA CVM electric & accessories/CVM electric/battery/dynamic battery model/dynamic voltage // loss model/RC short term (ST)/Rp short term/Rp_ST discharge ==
  bus : Inport
  Bus Selector : BusSelector  OutputSignals=gb.gb_cmd_gear,gb_spd_in_radps,ctrl.gb_line_press_bar
  Lookup : Lookup_n-D  NumberOfTableDimensions=10  BreakpointsForDimension1=LookupStructure.axis_1.breakpoints  BreakpointsForDimension2=LookupStructure.axis_2.breakpoints  BreakpointsForDimension3=LookupStructure.axis_3.breakpoints  BreakpointsForDimension4=LookupStructure.axis_4.breakpoints  BreakpointsForDimension5=LookupStructure.axis_5.breakpoints  BreakpointsForDimension6=LookupStructure.axis_6.breakpoints  BreakpointsForDimension7=LookupStructure.axis_7.breakpoints  BreakpointsForDimension8=LookupStructure.axis_8.breakpoints  BreakpointsForDimension9=LookupStructure.axis_9.breakpoints  BreakpointsForDimension10=LookupStructure.axis_10.breakpoints  IndexSearchMethod=Linear search  BeginIndexSearchUsingPreviousIndexResult=on  Table=LookupStructure.table  InternalRulePriority=Speed  RndMeth=Simplest  SupportTunableTableSize=on  MaximumIndicesForEachDimension=LookupStructure.table_size
  out : Outport
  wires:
  bus/1 -> Bus Selector/1
  Lookup/1 -> out/1

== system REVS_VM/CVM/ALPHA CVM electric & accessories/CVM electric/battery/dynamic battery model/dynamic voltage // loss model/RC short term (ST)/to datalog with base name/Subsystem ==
  Var : Inport
  Enable : EnablePort
  To Workspace : ToWorkspace  VariableName=datalog__battery__RC_ST_V  SampleTime=-1
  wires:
  Var/1 -> To Workspace/1

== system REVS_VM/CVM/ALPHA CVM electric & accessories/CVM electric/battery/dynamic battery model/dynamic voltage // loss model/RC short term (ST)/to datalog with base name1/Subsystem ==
  Var : Inport
  Enable : EnablePort
  To Workspace : ToWorkspace  VariableName=datalog__battery__RC_ST_Ohm  SampleTime=-1
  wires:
  Var/1 -> To Workspace/1

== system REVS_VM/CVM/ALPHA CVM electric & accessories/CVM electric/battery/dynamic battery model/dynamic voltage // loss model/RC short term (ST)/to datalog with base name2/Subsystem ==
  Var : Inport
  Enable : EnablePort
  To Workspace : ToWorkspace  VariableName=datalog__battery__RC_ST_Farad  SampleTime=-1
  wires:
  Var/1 -> To Workspace/1

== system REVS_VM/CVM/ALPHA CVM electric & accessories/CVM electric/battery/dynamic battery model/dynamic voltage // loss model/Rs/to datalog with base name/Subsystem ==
  Var : Inport
  Enable : EnablePort
  To Workspace : ToWorkspace  VariableName=datalog__battery__RS_V  SampleTime=-1
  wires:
  Var/1 -> To Workspace/1

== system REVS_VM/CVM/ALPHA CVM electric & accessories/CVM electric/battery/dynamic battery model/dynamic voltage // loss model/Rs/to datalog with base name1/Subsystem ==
  Var : Inport
  Enable : EnablePort
  To Workspace : ToWorkspace  VariableName=datalog__battery__RS_Ohm  SampleTime=-1
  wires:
  Var/1 -> To Workspace/1

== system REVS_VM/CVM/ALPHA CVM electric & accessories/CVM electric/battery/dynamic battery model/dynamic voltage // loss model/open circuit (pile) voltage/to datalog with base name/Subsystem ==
  Var : Inport
  Enable : EnablePort
  To Workspace : ToWorkspace  VariableName=datalog__battery__OCV_V  SampleTime=-1
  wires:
  Var/1 -> To Workspace/1

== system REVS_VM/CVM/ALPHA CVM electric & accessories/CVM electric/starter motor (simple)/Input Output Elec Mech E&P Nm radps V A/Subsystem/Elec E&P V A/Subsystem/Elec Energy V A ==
  volts_V : Inport
  curr_A : Inport  Port=2
  Gain : Gain  Gain=-1
  Integrator : Integrator  ZeroCross=off
  Integrator1 : Integrator  ZeroCross=off
  Integrator2 : Integrator  ZeroCross=off
  Mux : Mux  Inputs=2
  Neg : Fcn  Expr=u(1)*(u(1) <= 0)
  Pos : Fcn  Expr=u(1)*(u(1) >= 0)
  calc_Power_kW : Fcn  Expr=u(1)*u(2)/1000
  "total_kJ " : Outport
  "pos_kJ " : Outport  Port=2
  neg_kJ : Outport  Port=3
  pwr_kW : Outport  Port=4
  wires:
  curr_A/1 -> Mux/2
  volts_V/1 -> Mux/1
  Mux/1 -> calc_Power_kW/1
  Integrator/1 -> "total_kJ "/1
  Pos/1 -> Integrator1/1
  Neg/1 -> Integrator2/1
  Integrator2/1 -> Gain/1
  Integrator1/1 -> "pos_kJ "/1
  Gain/1 -> neg_kJ/1
  calc_Power_kW/1 -> Integrator/1, pwr_kW/1, Neg/1, Pos/1

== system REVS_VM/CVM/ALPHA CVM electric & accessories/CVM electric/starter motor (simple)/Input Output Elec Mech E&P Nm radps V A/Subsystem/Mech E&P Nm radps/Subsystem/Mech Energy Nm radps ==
  trq_Nm : Inport
  spd_radps : Inport  Port=2
  Gain : Gain  Gain=-1
  Integrator : Integrator  ZeroCross=off
  Integrator1 : Integrator  ZeroCross=off
  Integrator2 : Integrator  ZeroCross=off
  Mux : Mux  Inputs=2
  Neg : Fcn  Expr=u(1)*(u(1) <= 0)
  Pos : Fcn  Expr=u(1)*(u(1) >= 0)
  calc_Power_kW : Fcn  Expr=u(1)*u(2)/1000
  "total_kJ " : Outport
  "pos_kJ " : Outport  Port=2
  neg_kJ : Outport  Port=3
  pwr_kW : Outport  Port=4
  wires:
  calc_Power_kW/1 -> Pos/1, Neg/1, pwr_kW/1, Integrator/1
  Gain/1 -> neg_kJ/1
  Integrator1/1 -> "pos_kJ "/1
  Integrator2/1 -> Gain/1
  Neg/1 -> Integrator2/1
  Pos/1 -> Integrator1/1
  spd_radps/1 -> Mux/2
  trq_Nm/1 -> Mux/1
  Mux/1 -> calc_Power_kW/1
  Integrator/1 -> "total_kJ "/1

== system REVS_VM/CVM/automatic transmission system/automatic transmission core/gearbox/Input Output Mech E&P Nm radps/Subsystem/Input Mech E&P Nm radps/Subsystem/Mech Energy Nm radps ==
  trq_Nm : Inport
  spd_radps : Inport  Port=2
  Gain : Gain  Gain=-1
  Integrator : Integrator  ZeroCross=off
  Integrator1 : Integrator  ZeroCross=off
  Integrator2 : Integrator  ZeroCross=off
  Mux : Mux  Inputs=2
  Neg : Fcn  Expr=u(1)*(u(1) <= 0)
  Pos : Fcn  Expr=u(1)*(u(1) >= 0)
  calc_Power_kW : Fcn  Expr=u(1)*u(2)/1000
  "total_kJ " : Outport
  "pos_kJ " : Outport  Port=2
  neg_kJ : Outport  Port=3
  pwr_kW : Outport  Port=4
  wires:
  calc_Power_kW/1 -> Pos/1, Neg/1, pwr_kW/1, Integrator/1
  Gain/1 -> neg_kJ/1
  Integrator1/1 -> "pos_kJ "/1
  Integrator2/1 -> Gain/1
  Neg/1 -> Integrator2/1
  Pos/1 -> Integrator1/1
  spd_radps/1 -> Mux/2
  trq_Nm/1 -> Mux/1
  Mux/1 -> calc_Power_kW/1
  Integrator/1 -> "total_kJ "/1

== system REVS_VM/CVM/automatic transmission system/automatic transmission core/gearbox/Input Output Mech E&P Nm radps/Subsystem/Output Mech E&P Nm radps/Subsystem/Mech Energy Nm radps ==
  trq_Nm : Inport
  spd_radps : Inport  Port=2
  Gain : Gain  Gain=-1
  Integrator : Integrator  ZeroCross=off
  Integrator1 : Integrator  ZeroCross=off
  Integrator2 : Integrator  ZeroCross=off
  Mux : Mux  Inputs=2
  Neg : Fcn  Expr=u(1)*(u(1) <= 0)
  Pos : Fcn  Expr=u(1)*(u(1) >= 0)
  calc_Power_kW : Fcn  Expr=u(1)*u(2)/1000
  "total_kJ " : Outport
  "pos_kJ " : Outport  Port=2
  neg_kJ : Outport  Port=3
  pwr_kW : Outport  Port=4
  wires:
  calc_Power_kW/1 -> Pos/1, Neg/1, pwr_kW/1, Integrator/1
  Gain/1 -> neg_kJ/1
  Integrator1/1 -> "pos_kJ "/1
  Integrator2/1 -> Gain/1
  Neg/1 -> Integrator2/1
  Pos/1 -> Integrator1/1
  spd_radps/1 -> Mux/2
  trq_Nm/1 -> Mux/1
  Mux/1 -> calc_Power_kW/1
  Integrator/1 -> "total_kJ "/1

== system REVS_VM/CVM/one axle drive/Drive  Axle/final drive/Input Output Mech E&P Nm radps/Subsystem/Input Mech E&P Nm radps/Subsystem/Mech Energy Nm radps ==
  trq_Nm : Inport
  spd_radps : Inport  Port=2
  Gain : Gain  Gain=-1
  Integrator : Integrator  ZeroCross=off
  Integrator1 : Integrator  ZeroCross=off
  Integrator2 : Integrator  ZeroCross=off
  Mux : Mux  Inputs=2
  Neg : Fcn  Expr=u(1)*(u(1) <= 0)
  Pos : Fcn  Expr=u(1)*(u(1) >= 0)
  calc_Power_kW : Fcn  Expr=u(1)*u(2)/1000
  "total_kJ " : Outport
  "pos_kJ " : Outport  Port=2
  neg_kJ : Outport  Port=3
  pwr_kW : Outport  Port=4
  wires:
  calc_Power_kW/1 -> Pos/1, Neg/1, pwr_kW/1, Integrator/1
  Gain/1 -> neg_kJ/1
  Integrator1/1 -> "pos_kJ "/1
  Integrator2/1 -> Gain/1
  Neg/1 -> Integrator2/1
  Pos/1 -> Integrator1/1
  spd_radps/1 -> Mux/2
  trq_Nm/1 -> Mux/1
  Mux/1 -> calc_Power_kW/1
  Integrator/1 -> "total_kJ "/1

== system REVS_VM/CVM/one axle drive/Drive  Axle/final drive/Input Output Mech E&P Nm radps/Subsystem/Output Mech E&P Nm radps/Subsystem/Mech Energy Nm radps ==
  trq_Nm : Inport
  spd_radps : Inport  Port=2
  Gain : Gain  Gain=-1
  Integrator : Integrator  ZeroCross=off
  Integrator1 : Integrator  ZeroCross=off
  Integrator2 : Integrator  ZeroCross=off
  Mux : Mux  Inputs=2
  Neg : Fcn  Expr=u(1)*(u(1) <= 0)
  Pos : Fcn  Expr=u(1)*(u(1) >= 0)
  calc_Power_kW : Fcn  Expr=u(1)*u(2)/1000
  "total_kJ " : Outport
  "pos_kJ " : Outport  Port=2
  neg_kJ : Outport  Port=3
  pwr_kW : Outport  Port=4
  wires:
  calc_Power_kW/1 -> Pos/1, Neg/1, pwr_kW/1, Integrator/1
  Gain/1 -> neg_kJ/1
  Integrator1/1 -> "pos_kJ "/1
  Integrator2/1 -> Gain/1
  Neg/1 -> Integrator2/1
  Pos/1 -> Integrator1/1
  spd_radps/1 -> Mux/2
  trq_Nm/1 -> Mux/1
  Mux/1 -> calc_Power_kW/1
  Integrator/1 -> "total_kJ "/1
